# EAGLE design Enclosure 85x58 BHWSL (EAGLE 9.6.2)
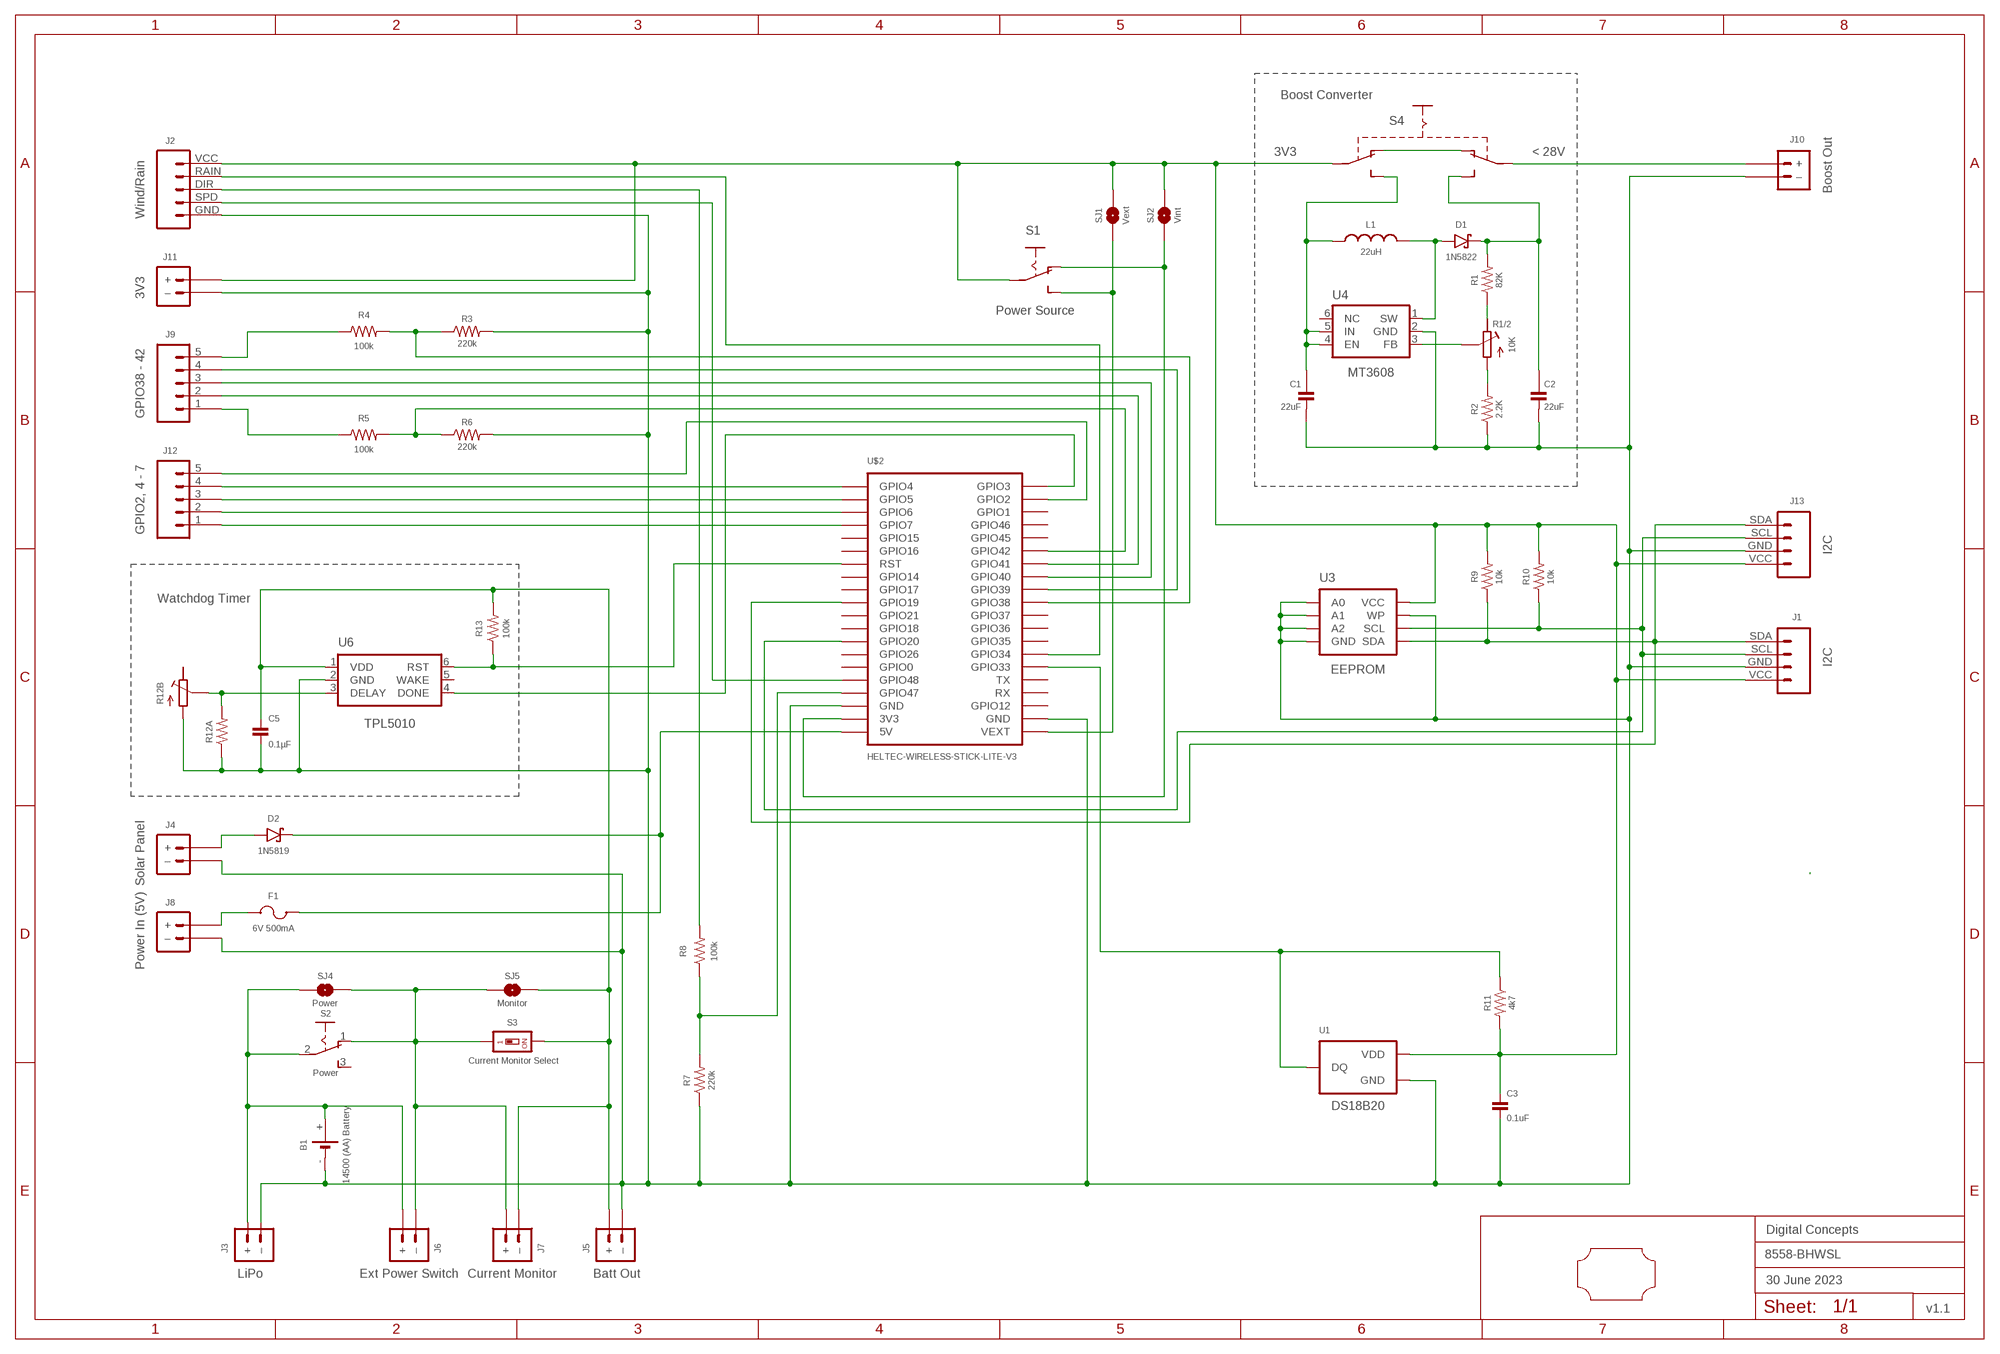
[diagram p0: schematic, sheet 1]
FRAME2 (A3L-LOC): DATE: 30 June 2023; OWNER: Digital Concepts; TITLE: 8558-BHWSL; VERSION: v1.1

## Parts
B1  14500 (AA) Battery  BATTERY-HOLDER-14500(AA)  [BATTERY-14500]
C1  22uF  CAPACITOR-1206  [C1206]
C2  22uF  CAPACITOR-1206  [C1206]
C3  0.1uF  CAPACITOR-0805  [C0805]
C5  0.1µF  CAPACITOR-0805  [C0805]
D1  1N5822  DIODE-SCHOTTKY-1N5822  [DIODE_SMB]
D2  1N5819  1N5819-SOD-123  [SOD-123]
F1  6V 500mA  MF-PSMF050X-2  [F0805]
J1  I2C  JST-PH2.0-4-VERTICAL-I2C  [JST-PH2.0-4-VERTICAL-I2C]
J2  Wind/Rain  JST-PH2.0-5-VERTICAL-WEATHER  [JST-PH2.0-5-WEATHER]
J3  LiPo  JST-PH2.0-2-MALE-HORIZONTALJST-PTH-2  [JST-PH2.0-2-HORIZONTAL]
J4  Solar Panel  JST-PH2.0-2-VERTICAL-POWER  [JST-PH2.0-2-VERTICAL-POWER]
J5  Batt Out  JST-GH1.25-2-HORIZONTAL-POWER  [JST-GH1.25-2-HORIZONTAL]
J6  Ext Power Switch  JST-PH2.0-2-DUAL-POWERJST-PTH-2  [JST-PH2.0-2-DUAL-POWER]
J7  Current Monitor  JST-PH2.0-2-HORIZONTAL-POWERJST-PTH-2  [JST-PH2.0-2-HORIZONTAL-POWER@1]
J8  Power In (5V)  JST-PH2.0-2-H-POWER  [JST-PH2.0-2-HORIZONTAL-POWER]
J9  GPIO38 - 42  JST-PH2.0-5-HORIZONTAL  [JST-PH2.0-5-HORIZONTAL]
J10  Boost Out  JST-PH2.0-2-H-POWER  [JST-PH2.0-2-HORIZONTAL-POWER]
J11  3V3  JST-PH2.0-2-H-POWER  [JST-PH2.0-2-HORIZONTAL-POWER]
J12  GPIO2, 4 - 7  JST-PH2.0-5-HORIZONTAL  [JST-PH2.0-5-HORIZONTAL]
J13  I2C  JST-PH2.0-4-HORIZONTAL-I2C  [JST-PH2.0-4-HORIZONTAL-I2C]
L1  22uH  INDUCTOR-CDRH104R/6D28L5038P  [CDRH104R+6D28]
R1  82K  RESISTORR0805  [R0805]
R1/2  10K  RESISTOR-TRIMM-BAOTER-HORIZONTAL  [RTRIM64P]
R2  2.2K  RESISTORR0805  [R0805]
R3  220k  RESISTORR0805  [R0805]
R4  100k  RESISTORR0805  [R0805]
R5  100k  RESISTORR0805  [R0805]
R6  220k  RESISTORR0805  [R0805]
R7  220k  RESISTORR0805  [R0805]
R8  100k  RESISTORR0805  [R0805]
R9  10k  RESISTORR0805  [R0805]
R10  10k  RESISTORR0805  [R0805]
R11  4k7  RESISTORR0805  [R0805]
R12A  RESISTORR0805  [R0805]
R12B  RESISTOR-TRIMM-33  [RTRIM3*3]
R13  100k  RESISTORR0805  [R0805]
S1  Power Source  SWITCH-SLIDE-SPDT-SMT  [SWITCH-SPDT-SMT]
S2  Power  SWITCH-SLIDE-SPDT  [SWITCH-SLIDE-SPDT]
S3  Current Monitor Select  SWITCH-DIP-SWS001  [SMD-001]
S4  SWITCH-SLIDE-DPDT-PTH-S  [SWITCH-DPDT-PTH]
SJ1  Vext  SJ  [SJ]
SJ2  Vint  SJ-V-1  [SJ-VIA-1]
SJ4  Power  SJ  [SJ]
SJ5  Monitor  SJ  [SJ]
U1  DS18B20  THERMOMETER-DS18B20  [TO-92]
U3  EEPROM  AT24CXX-EEPROM  [SOP-8]
U4  MT3608  [SOT-23-6@1]
U6  TPL5010  TPL5010DDCR  [SOT-23-6]
U$1  PCB-OUTLINE-85X58  [PROTO-28X18-OUTLINE]
U$2  HELTEC-WIRELESS-STICK-LITE-V3  [HELTEC-WIRELESS-STICK-LITE-V3]

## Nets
GND: B1.- C1.2 C2.2 C3.2 C5.2 J1.GND J2.GND J3.-(–) J4.-(–) J5.-(–) J8.-(–) J10.-(–) J11.-(–) J13.GND R2.1 R3.2 R6.2 R7.1 R12A.1 R12B.1(A) U1.1(GND) U3.P$1(A0) U3.P$2(A1) U3.P$3(A2) U3.P$4(GND) U3.P$7(WP) U4.2(GND) U6.2(GND) U$2.GND@18(GND) U$2.GND@22(GND)
N$1: D2.A J4.+
N$2: J2.DIR R8.2
N$3: R1.1 R1/2.3(E)
N$4: B1.+ J3.+ J6.+ S2.2(P) SJ4.2
N$5: D2.C F1.2 U$2.5V
N$6: D1.A L1.1 U4.1(SW)
N$7: R7.2 R8.1 U$2.GPIO47
N$8: J1.SCL J13.SCL R10.1 U3.P$6(SCL) U$2.GPIO20
N$9: J9.1 R5.1
N$10: J12.5 U$2.GPIO2
N$11: J1.SDA J13.SDA R9.1 U3.P$5(SDA) U$2.GPIO19
N$12: J2.SPD U$2.GPIO48
N$13: S1.P$1(O) SJ2.2 U$2.3V3
N$14: C5.1 J5.+ J7.-(–) R13.2 S3.2 SJ5.1 U6.1(VDD)
N$15: J12.4 U$2.GPIO4
N$16: J12.3 U$2.GPIO5
N$18: R11.1 U1.2(DQ) U$2.GPIO33
N$19: J12.2 U$2.GPIO6
N$20: C2.1 D1.C R1.2 S4.P$3(S1)
N$21: S1.P$2(S) SJ1.2 U$2.VEXT
N$22: J2.RAIN U$2.GPIO34
N$23: R1/2.1(A) R2.2
N$24: R1/2.2(S) U4.3(FB)
N$25: C1.1 L1.2 S4.P$6(S2) U4.4(EN) U4.5(IN)
N$26: S4.P$1(O1) S4.P$4(O2)
N$27: J10.+ S4.P$2(P1)
N$28: J12.1 U$2.GPIO7
N$29: J9.2 U$2.GPIO41
N$30: J9.3 U$2.GPIO40
N$31: J9.4 U$2.GPIO39
N$32: J9.5 R4.1
N$33: R3.1 R4.2 U$2.GPIO38
N$34: R5.2 R6.1 U$2.GPIO42
N$36: R12A.2 R12B.2(S) U6.3(DELAY)
N$37: R13.1 U6.6(RST) U$2.RST
N$38: U6.4(DONE) U$2.GPIO3
N$39: J6.-(–) J7.+ S2.1(O) S3.1 SJ4.1 SJ5.2
N$40: F1.1 J8.+
VCC: C3.1 J1.VCC J2.VCC J11.+ J13.VCC R9.2 R10.2 R11.2 S1.COMMON(P) S4.P$5(P2) SJ1.1 SJ2.1 SJ2.1@V U1.3(VDD) U3.P$8(VCC)
Unconnected: R12B.3(E) S2.3(S) U4.6(NC) U6.5(WAKE) U$2.GPIO0 U$2.GPIO1 U$2.GPIO12 U$2.GPIO14 U$2.GPIO15 U$2.GPIO16 U$2.GPIO17 U$2.GPIO18 U$2.GPIO21 U$2.GPIO26 U$2.GPIO35 U$2.GPIO36 U$2.GPIO37 U$2.GPIO45 U$2.GPIO46 U$2.RX U$2.TX

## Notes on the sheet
- Boost Converter
- 3V3 | < 28V
- Watchdog Timer

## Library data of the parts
B1 = digitalconcepts:BATTERY-HOLDER-14500(AA): 14500 (AA) battery holder
C1 C2 = digitalconcepts:CAPACITOR-1206: 1206 Capacitor
C3 C5 = digitalconcepts:CAPACITOR-0805: 0805 Capacitor
D1 = digitalconcepts:DIODE-SCHOTTKY-1N5822: 1N5822 Schottky Diode SMB
D2 = digitalconcepts:1N5819-SOD-123: 1N5819 Schottky Diode SOD-123
F1 = digitalconcepts:MF-PSMF050X-2: PTC Resettable Fuse
J1 = digitalconcepts:JST-PH2.0-4-VERTICAL-I2C: PH2.0 4P I2C Vertical Connector
J2 = digitalconcepts:JST-PH2.0-5-VERTICAL-WEATHER: PH2.0 5P Vertical Weather Connector
J3 = digitalconcepts:JST-PH2.0-2-MALE-HORIZONTAL: PH2.0 2P Right Angle PCB Connector; PROD_ID: CONN-09863; SKU: PRT-09914
J4 = digitalconcepts:JST-PH2.0-2-VERTICAL-POWER: JST PH2.0 2P PTH Connector (Power)
J5 = digitalconcepts:JST-GH1.25-2-HORIZONTAL-POWER: JST GH1.25 2P PTH Connector (Power)
J6 = digitalconcepts:JST-PH2.0-2-DUAL-POWER: JST PH2.0 2P PTH Dual-Side Connector (Power); PROD_ID: CONN-09863; SKU: PRT-09914
J7 = digitalconcepts:JST-PH2.0-2-HORIZONTAL-POWER: PH2.0 2P Right Angle PCB Connector; PROD_ID: CONN-09863; SKU: PRT-09914
J8 J10 J11 = digitalconcepts:JST-PH2.0-2-H-POWER: JST PH2.0 2P Right Angle Connector with power pin labelling
J9 J12 = digitalconcepts:JST-PH2.0-5-HORIZONTAL: PH2.0 5P Horizontal Connector
J13 = digitalconcepts:JST-PH2.0-4-HORIZONTAL-I2C: PH2.0 4P I2C Horizontal Connector
L1 = digitalconcepts:INDUCTOR-CDRH104R/6D28: Inductor; SPICEPREFIX: L
R1-R11 R12A R13 = digitalconcepts:RESISTOR: Resistor; SPICEPREFIX: R
R1/2 = digitalconcepts:RESISTOR-TRIMM-BAOTER-HORIZONTAL: Trimm Resistor - Horizontal BAOTER
R12B = digitalconcepts:RESISTOR-TRIMM-3*3: Trimm Resistor - 3*3 SMD
S1 = digitalconcepts:SWITCH-SLIDE-SPDT-SMT: Mini Sliding Switch SPDT SMT
S2 = digitalconcepts:SWITCH-SLIDE-SPDT: Mini Sliding Switch SPDT
S3 = digitalconcepts:SWITCH-DIP-SWS001: SMD Dip Switch 1 pol.
S4 = digitalconcepts:SWITCH-SLIDE-DPDT-PTH-S: Switch DPDT PTH-S
SJ1 SJ4 SJ5 = digitalconcepts:SJ: Solder Jumper
SJ2 = digitalconcepts:SJ-V-1: Solder Jumper with single Pad Via
U1 = digitalconcepts:THERMOMETER-DS18B20: Digital Thermometer -55C-125C TO92-3; AVAILABILITY: Bad; DESCRIPTION: Temperature Sensor Digital, Local -55°C ~ 125°C 12 b 8-uMAX; MF: Maxim Integrated; MP: DS18B20; PACKAGE: TO-92 Maxim Integrated; PRICE: None
U3 = digitalconcepts:AT24CXX-EEPROM: AT24Cxx EEPROM SOP-8
U4 = digitalconcepts:MT3608: MT3608 DC-DC Step-Up Voltage Converter
U6 = digitalconcepts:TPL5010DDCR: TPL5010 Nano-Power System Timer with Watchdog
U$1 = digitalconcepts:PCB-OUTLINE-85X58: PCB outline for 85 x 58 enclosure
U$2 = digitalconcepts:HELTEC-WIRELESS-STICK-LITE-V3: Heltec Wireless Stick Lite V3 MCU

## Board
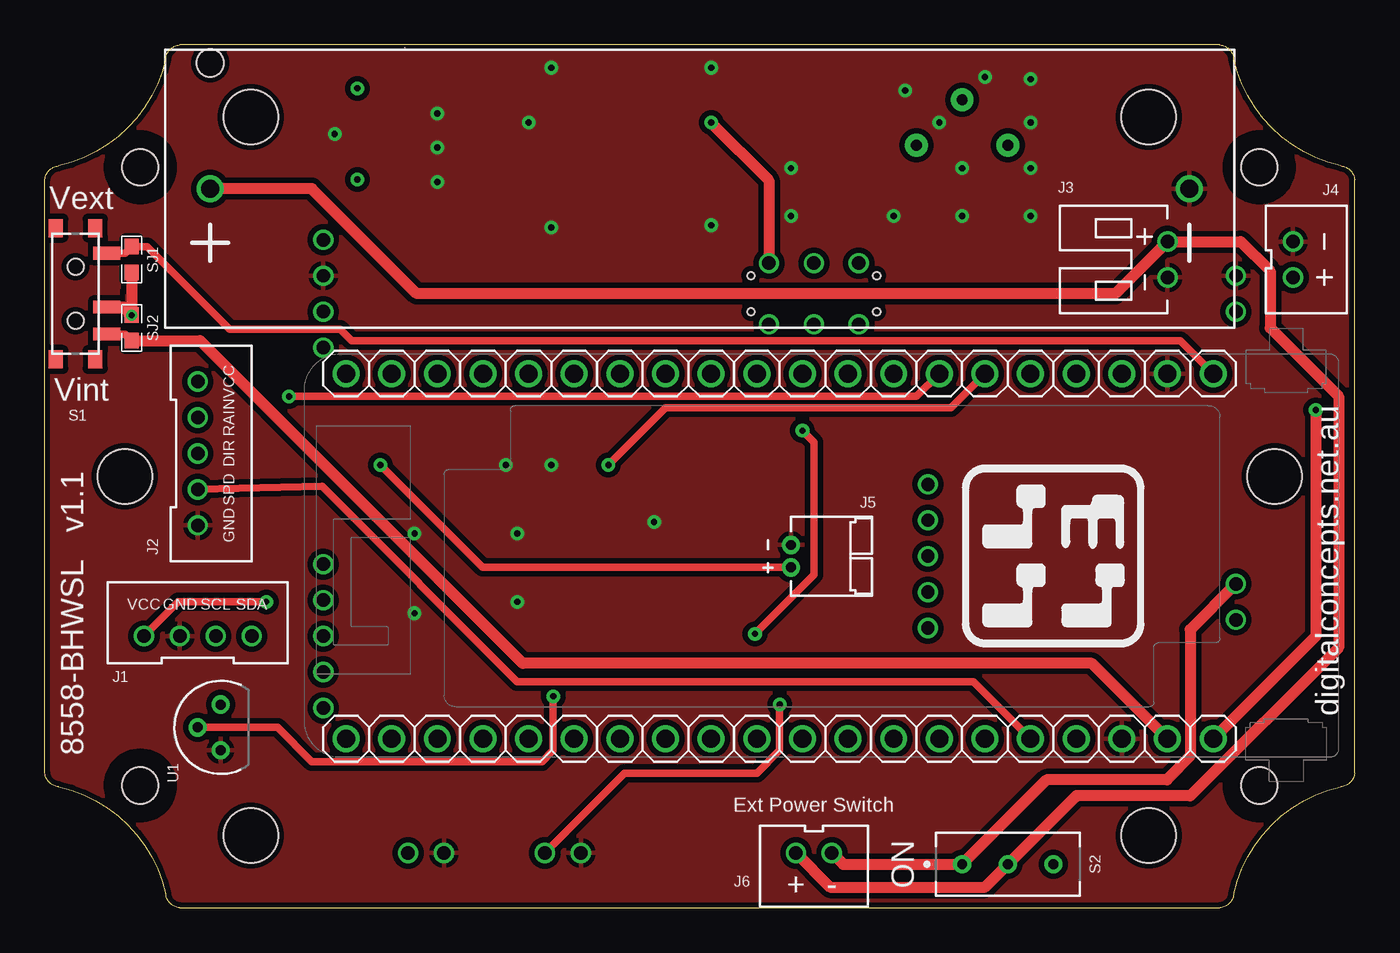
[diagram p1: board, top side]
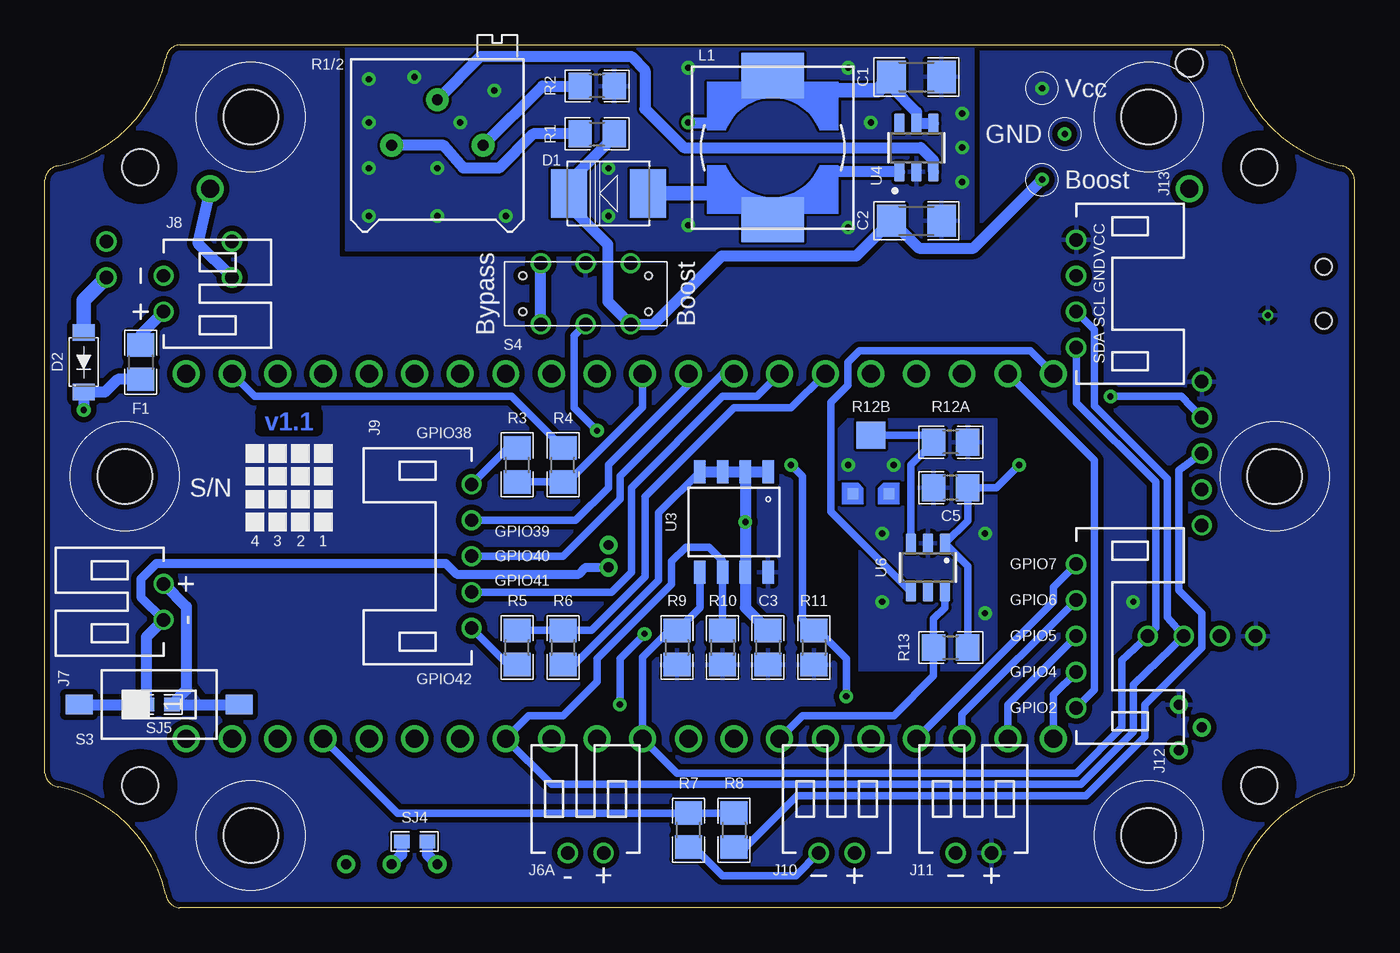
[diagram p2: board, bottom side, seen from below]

Size 72.9 x 48.01 mm. Coordinates in mm from the lower left corner, seen from the top.
Copper layers (1*16): Top 0.035mm / dielectric 1.5mm / Bottom 0.035mm
Design rules "default *": minimum track width 6mil, minimum drill 0.35mm, track to track 6mil, track to pad 6mil, pad to pad 6mil, via to via 6mil, smd to smd 6mil, copper to edge 6mil, drill to drill 6mil, minimum pad ring 1mil, minimum via ring 8mil, stop-mask expansion 4mil, vias tented up to drill 0mil, thermal gap 10mil

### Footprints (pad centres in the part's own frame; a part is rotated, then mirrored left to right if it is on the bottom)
BATTERY-14500 = drill 1: + -27.25,0; - 27.25,0 | hole 1.524: -27.25,7
C1206 = smd 1.6 x 1.8: 1 -1.4,0; 2 1.4,0
C0805 = smd 1.3 x 1.5: 1 -0.95,0; 2 0.95,0
DIODE_SMB = smd 2 x 2.7: A 2.2,0; C -2.2,0
SOD-123 = smd 0.91 x 1.22: A -1.65,0; C 1.65,0
F0805 = smd 1.3 x 1.5: 1 -0.95,0; 2 0.95,0
JST-PH2.0-4-VERTICAL-I2C = drill 0.75: GND 1,0; SCL -1,0; SDA -3,0; VCC 3,0
JST-PH2.0-5-WEATHER = drill 0.75: DIR 0,0; GND -4,0; RAIN 2,0; SPD -2,0; VCC 4,0
JST-PH2.0-2-HORIZONTAL = drill 0.75: + 1,0; - -1,0
JST-PH2.0-2-VERTICAL-POWER = drill 0.75: + -1,0; - 1,0
JST-GH1.25-2-HORIZONTAL = drill 0.55 pad 1.016: + -0.625,0; - 0.625,0
JST-PH2.0-2-DUAL-POWER = drill 0.75: + 1,0; - -1,0
JST-PH2.0-2-HORIZONTAL-POWER@1 = drill 0.75: + 1,0; - -1,0
JST-PH2.0-2-HORIZONTAL-POWER = drill 0.75: + 1,0; - -1,0
JST-PH2.0-5-HORIZONTAL = drill 0.75: 1 4,0; 2 2,0; 3 0,0; 4 -2,0; 5 -4,0
JST-PH2.0-4-HORIZONTAL-I2C = drill 0.75: GND -1,0; SCL 1,0; SDA 3,0; VCC -3,0
CDRH104R+6D28 = smd 2.5 x 3.5: 1 -4,0; 2 4,0
R0805 = smd 1.3 x 1.5: 1 -0.95,0; 2 0.95,0
RTRIM64P = drill 0.61 pad 1.27: 1 0,-2.54; 2 2.54,0; 3 0,2.54
RTRIM3*3 = smd 0.6 x 0.6: 1 -1,-1.6; 3 1,-1.6 | smd 1.6 x 1.5: 2 0,1.65
SWITCH-SPDT-SMT = smd 0.7 x 1.5: COMMON 0.75,1.75; P$1 2.25,1.75; P$2 -2.25,1.75 | smd 1 x 0.8: GND@1 3.65,-1.1; GND@2 3.65,1.1; GND@3 -3.65,1.1; GND@4 -3.65,-1.1 | hole 0.9: -1.5,0; 1.5,0
SWITCH-SLIDE-SPDT = drill 0.55 pad 1.016: 1 -2.54,0; 2 0,0; 3 2.54,0
SMD-001 = smd 1.1 x 1.5: 1 0,-4.45; 2 0,4.45
SWITCH-DPDT-PTH = drill 0.75: P$1 -1.7,2.5; P$2 -1.7,0; P$3 -1.7,-2.5; P$4 1.7,2.5; P$5 1.7,0; P$6 1.7,-2.5 | hole 0.42: 1,3.5; -1,3.5; 1,-3.5; -1,-3.5
SJ = smd 0.864 x 0.762: 1 -0.711,0; 2 0.711,0
SJ-VIA-1 = smd 0.864 x 0.762: 1 -0.711,0; 2 0.711,0 | drill 0.35 pad 0.61: 1@V -0.711,0
TO-92 = drill 0.55 pad 1.016: 1 -1.27,0; 2 0,1.27; 3 1.27,0
SOP-8 = smd 0.635 x 1.27: P$1 -1.905,-2.794; P$2 -0.635,-2.794; P$3 0.635,-2.794; P$4 1.905,-2.794; P$5 1.905,2.794; P$6 0.635,2.794; P$7 -0.635,2.794; P$8 -1.905,2.794
SOT-23-6@1 = smd 1.1 x 0.6: 1 -1.35,0.95; 2 -1.35,0; 3 -1.35,-0.95; 4 1.35,-0.95; 5 1.35,0; 6 1.35,0.95
SOT-23-6 = smd 1.1 x 0.6: 1 -1.35,0.95; 2 -1.35,0; 3 -1.35,-0.95; 4 1.35,-0.95; 5 1.35,0; 6 1.35,0.95
PROTO-28X18-OUTLINE = hole 2.032: -31.14,17.196; -31.14,-17.196; 31.14,-17.196; 31.14,17.196 | hole 3.048: -24.994,19.99; -32.004,0; -24.994,-19.99; 24.994,-19.99; 32.004,0; 24.994,19.99
HELTEC-WIRELESS-STICK-LITE-V3 = drill 1: 3V3 0,45.72; 5V 0,48.26; GND@18 0,43.18; GND@22 -20.32,45.72; GPIO0 0,35.56; GPIO1 -20.32,5.08; GPIO2 -20.32,2.54; GPIO3 -20.32,0; GPIO4 0,0; GPIO5 0,2.54; GPIO6 0,5.08; GPIO7 0,7.62; GPIO12 -20.32,43.18; GPIO14 0,17.78; GPIO15 0,10.16; GPIO16 0,12.7; GPIO17 0,20.32; GPIO18 0,27.94; GPIO19 0,22.86; GPIO20 0,30.48; GPIO21 0,25.4; GPIO26 0,33.02; GPIO33 -20.32,35.56; GPIO34 -20.32,33.02; GPIO35 -20.32,30.48; GPIO36 -20.32,27.94; GPIO37 -20.32,25.4; GPIO38 -20.32,22.86; GPIO39 -20.32,20.32; GPIO40 -20.32,17.78; GPIO41 -20.32,15.24; GPIO42 -20.32,12.7; GPIO45 -20.32,10.16; GPIO46 -20.32,7.62; GPIO47 0,40.64; GPIO48 0,38.1; RST 0,15.24; RX -20.32,40.64; TX -20.32,38.1; VEXT -20.32,48.26

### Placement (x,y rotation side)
B1  36.45,40.01 0 top
C1  24.38,46.23 0 bottom
C2  24.38,38.23 0 bottom
C3  32.64,14.48 90 bottom
C5  22.48,23.37 180 bottom
D1  41.53,39.75 0 bottom
D2  70.74,30.35 270 bottom
F1  67.56,30.35 270 bottom
J1  8.51,15.11 180 top
J2  8.51,25.27 90 top
J3  62.48,36.07 90 top
J4  69.47,36.07 90 top
J5  41.53,19.56 90 top
J6  42.8,3.05 0 bottom
J7  66.29,17.02 90 bottom
J8  66.29,34.16 270 bottom
J9  49.15,19.56 270 bottom
J10  28.83,3.05 0 bottom
J11  21.21,3.05 0 bottom
J12  15.49,15.11 90 bottom
J13  15.49,34.16 270 bottom
L1  32.38,42.29 90 bottom
R1  42.16,43.05 0 bottom
R1/2  51.05,42.42 90 bottom
R2  42.16,45.72 180 bottom
R3  44.07,24.64 90 bottom
R4  46.61,24.64 270 bottom
R5  46.61,14.48 90 bottom
R6  44.07,14.48 270 bottom
R7  37.08,4.32 90 bottom
R8  34.54,4.32 270 bottom
R9  37.72,14.48 270 bottom
R10  35.18,14.48 270 bottom
R11  30.1,14.48 270 bottom
R12A  22.48,25.91 180 bottom
R12B  26.92,24.64 0 bottom
R13  22.48,14.48 0 bottom
S1  1.7,34.16 270 top
S2  53.59,2.41 0 top
S3  66.55,11.3 90 bottom
S4  42.8,34.16 90 bottom
SJ1  4.83,36.07 90 top
SJ2  4.83,32.26 270 top
SJ4  52.32,3.68 180 bottom
SJ5  66.55,11.3 0 bottom
U1  9.78,10.03 90 top
U3  34.54,21.46 180 bottom
U4  24.38,42.29 90 bottom
U6  23.75,18.92 270 bottom
U$1  36.45,24 0 top
U$2  16.76,9.4 270 top

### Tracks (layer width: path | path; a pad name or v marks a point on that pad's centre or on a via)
$X1
  cutout Bottom: 67.59,43.23 arc180 67.59,39.17 arc180
$X2
  cutout Bottom: 67.59,8.84 arc180 67.59,4.78 arc180
$X3
  cutout Bottom: 5.31,8.84 arc180 5.31,4.78 arc180
$X4
  cutout Bottom: 5.31,43.23 arc180 5.31,39.17 arc180
$X5
  cutout Top: 5.31,43.23 arc180 5.31,39.17 arc180
$X6
  cutout Top: 67.59,43.23 arc180 67.59,39.17 arc180
$X7
  cutout Top: 67.59,8.84 arc180 67.59,4.78 arc180
$X8
  cutout Top: 5.31,8.84 arc180 5.31,4.78 arc180
GND  (via drill 0.35)
  Bottom 0.406: J10.- 31.1,1.78 35.18,1.78 36.77,3.37 R7.1 | U$2.GND@22 61.21,28.45 46.93,28.45 R3.2 | R6.2 43.43,13.53 38.73,18.23 38.73,21.97 U3.P$4
  Bottom 0.61: U3.P$4 U3.P$3 U3.P$2 | U3.P$2 U3.P$1 | B1.- 64.39,36.97 J3.- | C3.2 33.91,16.7 U3.P$7 v33.91,21.46 U3.P$2
  other vias: 21.84,44.2 26.92,43.69 37.08,37.97 37.08,46.74 47.88,45.47 52.32,46.23 41.53,38.48 47.24,38.48 51.05,38.48 51.05,41.15 54.86,38.48 54.86,41.15 54.86,46.1 21.84,40.39 49.78,43.69 54.86,43.69 28.19,37.85 41.53,41.15 16.13,43.05 21.84,42.29 28.19,46.74 28.19,24.64 25.65,24.64 20.57,20.83 20.57,16.38 26.29,20.83 26.29,17.02
  pour Top (isolate 0.305, rank 2): -2.08,49.93 -2.08,-1.97 74.92,-1.97 74.92,49.93
  pour Bottom (rank 2): 21.21,48.13 21.21,36.58 56.13,36.58 56.13,48.13
  pour Bottom: 27.56,13.21 19.94,13.21 19.94,27.18 28.19,27.18 28.83,26.54 28.83,22.1 27.56,20.83
N$1
  Bottom 0.813: D2.A 70.74,33.8 J4.+
N$2
  Bottom 0.406: R8.2 33.91,3.37 31.04,6.24 14.97,6.24 11.68,9.53 11.68,11.3 8.51,14.48 8.51,16.38 9.78,17.65 9.78,24.33 J2.DIR
N$3
  Bottom 0.61: R1.1 45.72,43.05 47.62,41.15 49.6,41.15 50.69,42.42 R1/2.3
N$4
  Top 0.61: B1.+ 14.86,40.01 20.7,34.16 59.58,34.16 J3.+ 66.56,37.07 68.2,35.43 68.2,32.26 72.01,28.45 72.01,14.48 63.75,6.22 57.48,6.22 | 57.48,6.22 57.42,6.24 S2.2 52.32,1.14 43.7,1.14 J6.+ | 57.48,6.22
  Bottom 0.61: SJ4.2 53.03,2.97 S2.2
N$5  (via drill 0.35)
  Top 0.61: U$2.5V 70.74,15.11 v70.74,27.69
  Bottom 0.61: v70.74,27.69 D2.C 69.55,28.7 68.84,29.4 F1.2
N$6
  Bottom 0.61: L1.1 31.75,38.29 29.1,40.94 U4.1
  Bottom 0.813: D1.A 34.54,39.75 33.08,38.29 L1.1
N$7
  Bottom 0.406: R8.1 R7.2 53.27,5.27 U$2.GPIO47
N$8
  Bottom 0.406: J13.SCL 14.48,32.15 14.48,27.94 10.41,23.88 10.41,16.16 J1.SCL 12.32,12.41 12.32,9.78 15.24,6.86 44.7,6.86 U$2.GPIO20 45.97,10.67 44.07,10.67 42.16,12.57 42.16,13.84 38.01,18 38.01,19.27 37.21,20.07 35.94,20.07 35.18,19.3 U3.P$6 R10.1
N$9
  Bottom 0.406: J9.1 47.12,13.53 R5.1
N$10
  Bottom 0.406: J12.5 14.48,12.13 14.48,24.89 U$2.GPIO2
N$11
  Bottom 0.406: J13.SDA 15.49,28.1 11.05,23.7 11.05,15.57 J1.SDA 12.95,13.78 12.95,10.03 15.49,7.49 37.72,7.49 U$2.GPIO19 39.62,13.93 38.12,15.43 R9.1 36.45,16.7 U3.P$5
N$12
  Top 0.406: J2.SPD 15.42,23.44 26.29,12.57 51.69,12.57 U$2.GPIO48
N$13
  Top 0.406: SJ2.2 4.46,31.91 S1.P$1
  Top 0.61: SJ2.2 8.64,31.55 26.59,13.59 58.28,13.59 U$2.3V3
N$14  (via drill 0.35)
  Top 0.406: J5.+ 24.37,18.93 v18.67,24.64
  Bottom 0.406: R13.2 21.53,19 U6.1 21.53,21.54 C5.1 19.94,23.37 v18.67,24.64
  Bottom 0.508: J7.- 67.56,17.29 67.56,18.29 66.69,19.16 50.59,19.16 49.98,18.56 43.17,18.56 42.8,18.93 J5.+
  Bottom 0.61: S3.2 SJ5.1 67.26,15.05 J7.-
N$15
  Bottom 0.406: J12.4 16.76,11.84 U$2.GPIO4
N$16
  Bottom 0.406: J12.3 19.3,11.3 U$2.GPIO5
N$18  (via drill 0.35)
  Top 0.406: U$2.GPIO33 50.42,27.81 34.54,27.81 v31.37,24.64 | v28.29,11.76 28.29,8.76 27.66,8.13 14.86,8.13 12.95,10.03 U1.2
  Bottom 0.406: v31.37,24.64 30.73,24 30.73,16.06 R11.1 29.88,15.43 28.29,13.84 v28.29,11.76
N$19
  Bottom 0.406: J12.2 21.84,10.76 U$2.GPIO6
N$20  (via drill 0.35)
  Bottom 0.61: v17.4,40.51 21.21,36.7 24.26,36.7 C2.1 27.74,36.27 35.22,36.27 39.03,32.46 S4.P$3 41.57,33.73 41.57,36.91 43.73,39.07 D1.C 43.73,40.39 41.21,42.91 R1.2
N$21
  Top 0.406: S1.P$2 4.46,36.41 SJ1.2 5.7,36.78 10.29,32.18 16.42,32.18 17.06,31.55 63.2,31.55 U$2.VEXT
N$22  (via drill 0.35)
  Top 0.406: U$2.GPIO34 48.51,28.45 v13.59,28.45
  Bottom 0.406: J2.RAIN 9.65,28.45 v13.59,28.45
N$23
  Bottom 0.61: R1/2.1 45.21,45.72 R2.2
N$24
  Bottom 0.61: R1/2.2 48.64,47.37 40.26,47.37 39.5,46.61 39.5,44.45 37.34,42.29 24.15,42.29 23.43,41.58 U4.3
N$25  (via drill 0.35)
  Top 0.61: v37.08,43.69 40.3,40.47 S4.P$6
  Bottom 0.61: C1.1 25.78,45.67 24.38,44.27 U4.5 U4.4 | v37.08,43.69 35.81,43.69 33.21,46.29 L1.2
  Bottom 0.813: C1.1 26.53,45.48 31.58,45.48 L1.2
N$26
  Bottom 0.61: S4.P$1 S4.P$4
N$27  (via drill 0.35)
  Top 0.406: J10.+ 32.27,7.49 39.62,7.49 40.89,8.76 v40.89,11.3 | v42.16,26.54 42.8,25.91 42.8,18.52 v39.52,15.24
  Bottom 0.406: v40.89,11.3 40.89,13.84 39.52,15.22 v39.52,15.24 | v42.16,26.54 43.43,27.81 43.43,31.83 S4.P$2
N$28
  Bottom 0.406: J12.1 16.76,17.84 16.76,17.02 U$2.GPIO7
N$29
  Bottom 0.406: J9.2 41.37,17.56 40.26,18.67 40.26,23.37 35.18,28.45 33.27,28.45 U$2.GPIO41
N$30
  Bottom 0.406: J9.3 44.07,19.56 40.89,22.73 40.89,24 35.18,29.72 U$2.GPIO40
N$31
  Bottom 0.406: U$2.GPIO39 37.08,29.11 41.53,24.64 41.53,23.37 43.36,21.56 J9.4
N$32
  Bottom 0.406: J9.5 47.12,25.59 R4.1
N$33
  Bottom 0.406: U$2.GPIO38 39.62,27.85 43.79,23.69 R3.1 R4.2
N$34
  Bottom 0.406: U$2.GPIO42 31.37,27.81 34.54,27.81 39.5,22.86 39.5,18.41 42.48,15.43 R6.1 R5.2
N$36
  Bottom 0.406: R12B.2 23.81,26.29 R12A.2 24.7,24.64 U6.3
N$37
  Bottom 0.406: U6.6 22.8,16.7 23.43,16.07 R13.1 23.43,12.89 25.65,10.67 30.73,10.67 U$2.RST
N$38
  Bottom 0.406: U$2.GPIO3 18.03,30.99 27.56,30.99 28.19,30.35 28.19,29.08 29.14,28.13 29.14,22.02 U6.4
N$39
  Top 0.61: J7.+ 63.75,15.48 63.75,8.46 62.46,7.11 55.75,7.11 S2.1 44.43,2.41 J6.-
  Bottom 0.61: J7.+ 65.02,16.75 65.02,12.12 SJ5.2 S3.1 | SJ4.1 51.61,2.97 S2.1
  pour Bottom: 65.85,11.3 65.02,12.12 64.39,11.3
N$40
  Bottom 0.61: J8.+ 67.56,31.89 F1.1
VCC  (via drill 0.35)
  Top 0.406: J1.VCC 7.41,17.02 v12.32,17.02
  Top 0.61: S1.COMMON 4.38,33.41 SJ2.1@V SJ1.1
  other vias: 17.4,45.59
  pour Bottom (isolate 0.305, rank 5): -1.08,48.93 -1.08,-0.97 73.92,-0.97 73.92,48.93
  pour Top: 4.22,33.46 4.7,33.93 4.7,32.98

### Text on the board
Bottom: v1.1
tPlace: digitalconcepts.net.au | 8558-BHWSL v1.1
bPlace: S/N | 1 | 2 | 3 | 4
tNames: Vext | Vint | ON
bNames: Vcc | GND | Boost | Boost | Bypass | GPIO38 | GPIO39 | GPIO40 | GPIO7 | GPIO41 | GPIO6 | GPIO5 | GPIO4 | GPIO42 | GPIO2 | J6A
